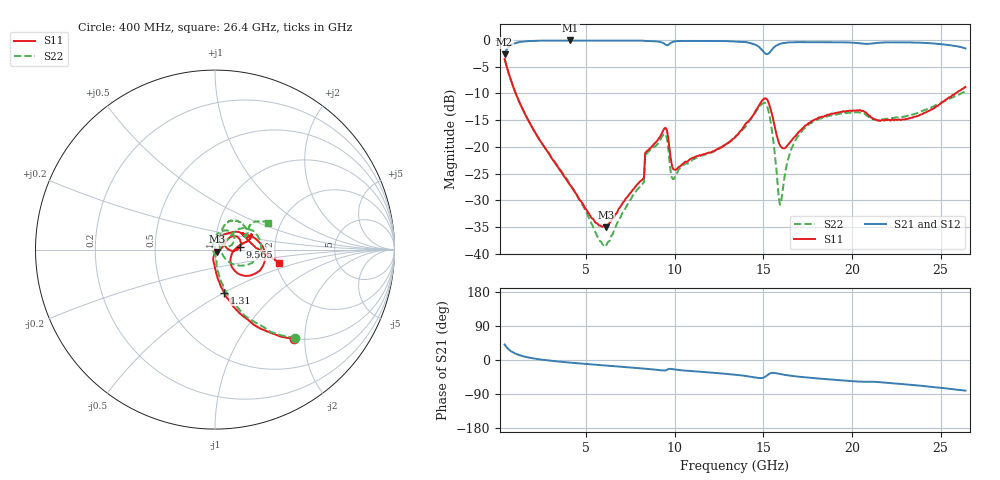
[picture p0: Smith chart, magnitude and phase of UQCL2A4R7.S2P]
! AVX Corporation
! Date:  10/27/06
! Part No:  UQCL2A4R7
! Description:  Ultra Low ESR Microwave capacitors
! Mounting Orientation:  Horizontal
# GHZ S DB R 50
! Freq  |S11|  S11 Ph  |S21|  S21 Ph  |S12|  S12 Ph  |S22|  S22 Ph
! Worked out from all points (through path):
!   401 points, 400 MHz to 26.4 GHz, reference 50 ohm
!   highest |S21| = -0.09 dB at 4.105 GHz (marker M1); lowest = -2.7 dB at 400 MHz (marker M2)
!   group delay of S21, straight-line fit = 9.08 ps
!   lowest |S11| = -35.0 dB at 6.12 GHz (marker M3), VSWR 1.04, Z = 51.4 - j1.14 ohm
!   |S11| at or under -10 dB: 1.028 GHz to 25.84 GHz (24.81 GHz wide, 185 % of centre)
!   |S22| runs from -38.6 to -3.5 dB; largest |S21 - S12| = 0.0089
!   S11 on the Smith chart (normalised r, x): 400 MHz: 0.99, -1.77; 1.31 GHz: 0.98, -0.50; 9.565 GHz: 1.33, +0.04; 26.4 GHz: 2.07, -0.35
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0.4  -3.55 -48.6  -2.67 41.0  -2.67 41.0  -3.53 -47.7
0.79  -7.85 -66.9  -0.88 22.3  -0.88 22.2  -7.89 -65.8
1.31  -12.20 -78.0  -0.36 11.7  -0.36 11.8  -12.18 -75.0
4.105  -27.21 -101.6  -0.09 -7.0  -0.09 -7.0  -26.95 -83.9
4.755  -30.37 -97.0  -0.09 -9.6  -0.10 -9.6  -30.63 -90.6
6.12  -35.04 -38.7  -0.10 -14.7  -0.10 -14.6  -38.60 -170.9
8.135  -26.26 24.1  -0.13 -22.0  -0.14 -21.9  -27.07 89.8
8.46  -20.71 39.8  -0.20 -23.5  -0.19 -23.5  -21.10 81.5
9.11  -18.38 37.9  -0.32 -26.4  -0.32 -26.4  -19.10 67.8
9.565  -17.00 5.8  -1.00 -25.8  -1.00 -25.7  -18.57 24.3
9.955  -24.26 19.6  -0.30 -24.6  -0.29 -24.6  -26.00 43.5
13.4  -18.25 48.9  -0.30 -39.0  -0.31 -39.0  -18.22 41.2
14.57  -13.20 20.3  -0.92 -46.3  -0.93 -46.2  -13.50 33.4
15.155  -10.97 -18.4  -2.62 -42.5  -2.60 -42.4  -12.03 -5.5
15.415  -13.00 -41.0  -2.11 -34.6  -2.10 -34.7  -15.37 -31.9
15.87  -19.19 -37.8  -0.81 -36.3  -0.81 -36.2  -29.51 -15.6
16  -20.03 -28.9  -0.67 -37.5  -0.67 -37.5  -30.19 31.6
16.65  -18.58 3.6  -0.43 -42.2  -0.43 -42.1  -19.88 70.6
17.755  -15.12 13.7  -0.41 -47.5  -0.40 -47.4  -15.45 64.9
20.355  -13.23 22.6  -0.60 -56.9  -0.58 -56.9  -13.52 34.9
22.11  -14.97 30.8  -0.45 -60.7  -0.44 -60.6  -14.65 25.4
26.4  -8.79 -11.6  -1.58 -80.8  -1.59 -81.2  -9.61 27.1
